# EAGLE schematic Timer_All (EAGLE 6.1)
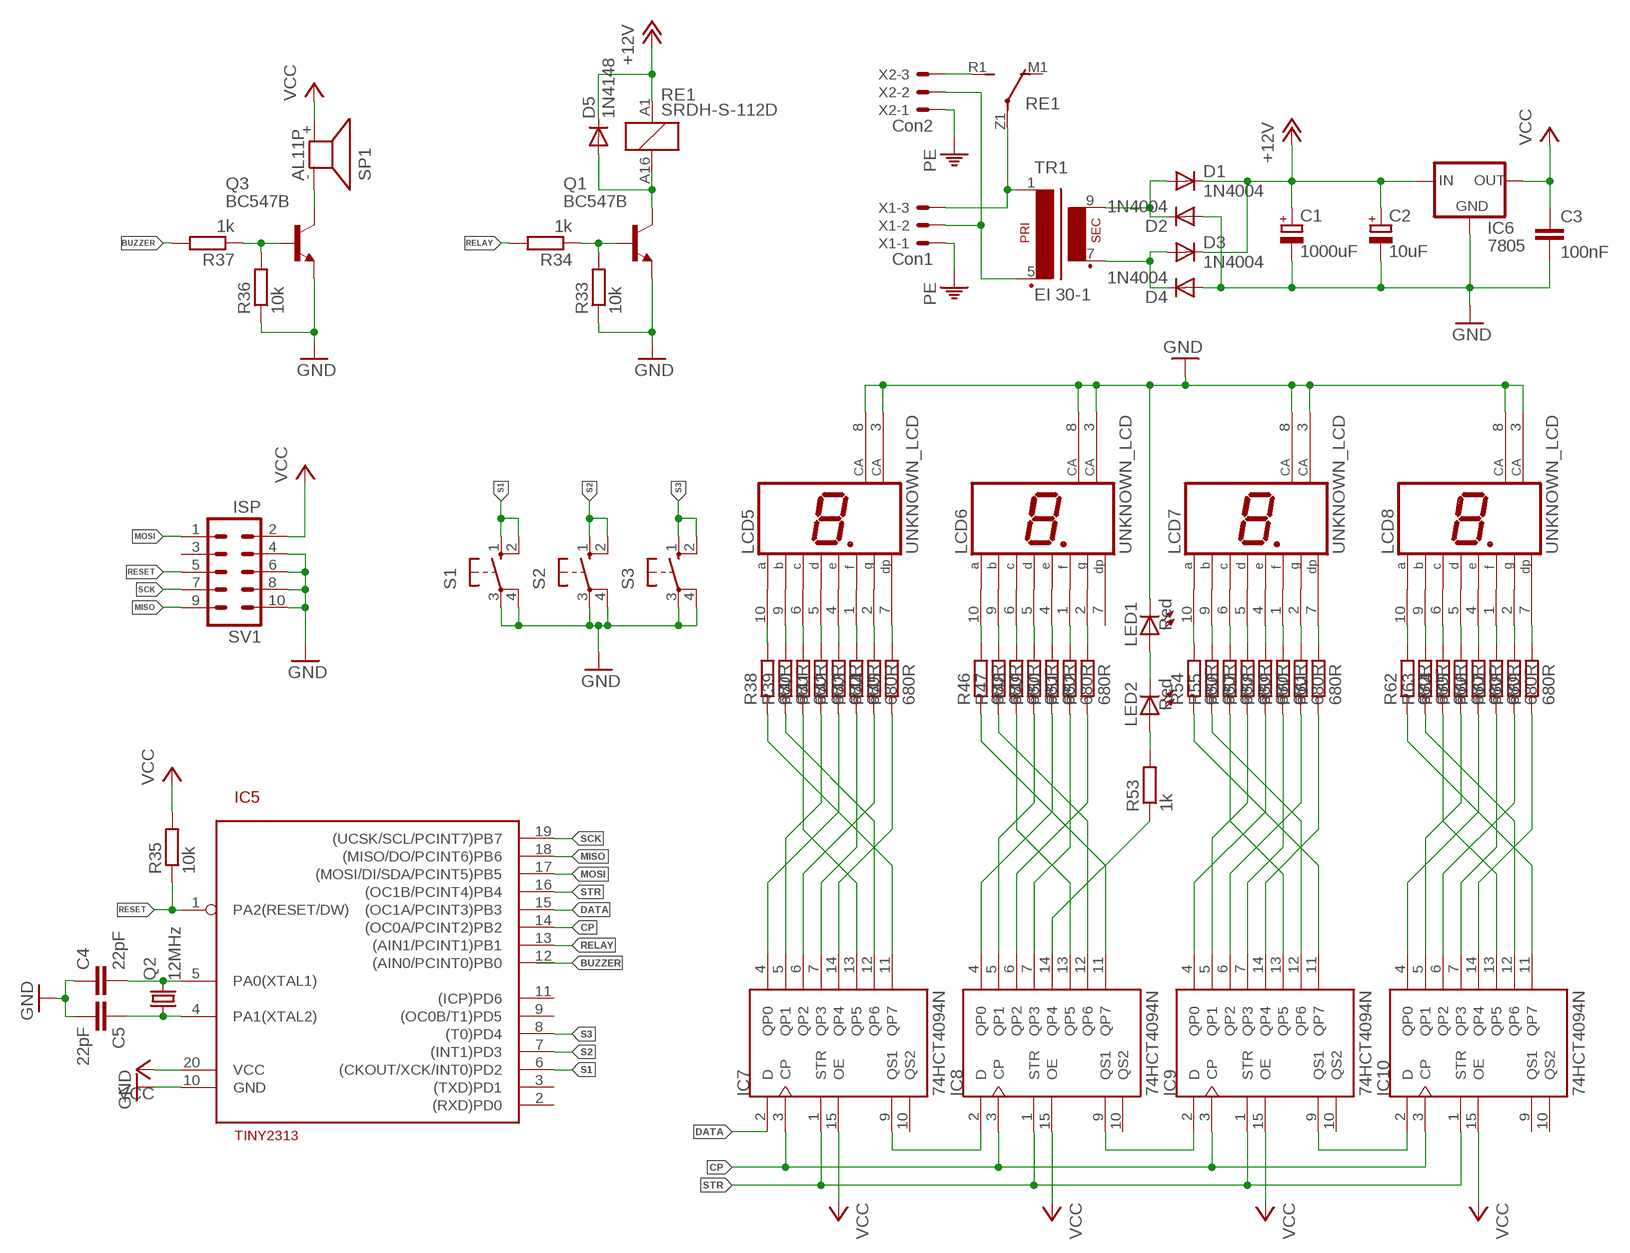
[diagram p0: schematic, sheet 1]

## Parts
C1  1000uF  CPOL-EUTT5D10  [TT5D10]
C2  10uF  CPOL-EUE2.5-5  [E2,5-5]
C3  100nF  C-EU050-025X075  [C050-025X075]
C4  22pF  C-EU025-025X050  [C025-025X050]
C5  22pF  C-EU025-025X050  [C025-025X050]
D1  1N4004  [DO41-10]
D2  1N4004  [DO41-10]
D3  1N4004  [DO41-10]
D4  1N4004  [DO41-10]
D5  1N4148  1N4148DO35-10  [DO35-10]
IC5  TINY2313  [DIL20]
IC6  7805  78XXL  [78XXL]
IC7  74HCT4094N  [DIL16]
IC8  74HCT4094N  [DIL16]
IC9  74HCT4094N  [DIL16]
IC10  74HCT4094N  [DIL16]
LCD5  UNKNOWN_LCD  [CA-MOJ]
LCD6  UNKNOWN_LCD  [CA-MOJ]
LCD7  UNKNOWN_LCD  [CA-MOJ]
LCD8  UNKNOWN_LCD  [CA-MOJ]
LED1  Red  LED3MM  [LED3MM]
LED2  Red  LED3MM  [LED3MM]
Q1  BC547B  [TO92]
Q2  12MHz  CRYSTALHC49S  [HC49/S]
Q3  BC547B  [TO92]
R33  10k  R-EU_0207/10  [0207/10]
R34  1k  R-EU_0207/10  [0207/10]
R35  10k  R-EU_0207/10  [0207/10]
R36  10k  R-EU_0207/10  [0207/10]
R37  1k  R-EU_0207/10  [0207/10]
R38  680R  R-EU_R0805  [R0805]
R39  680R  R-EU_R0805  [R0805]
R40  680R  R-EU_R0805  [R0805]
R41  680R  R-EU_R0805  [R0805]
R42  680R  R-EU_R0805  [R0805]
R43  680R  R-EU_R0805  [R0805]
R44  680R  R-EU_R0805  [R0805]
R45  680R  R-EU_R0805  [R0805]
R46  680R  R-EU_R0805  [R0805]
R47  680R  R-EU_R0805  [R0805]
R48  680R  R-EU_R0805  [R0805]
R49  680R  R-EU_R0805  [R0805]
R50  680R  R-EU_R0805  [R0805]
R51  680R  R-EU_R0805  [R0805]
R52  680R  R-EU_R0805  [R0805]
R53  1k  R-EU_0207/10  [0207/10]
R54  680R  R-EU_R0805  [R0805]
R55  680R  R-EU_R0805  [R0805]
R56  680R  R-EU_R0805  [R0805]
R57  680R  R-EU_R0805  [R0805]
R58  680R  R-EU_R0805  [R0805]
R59  680R  R-EU_R0805  [R0805]
R60  680R  R-EU_R0805  [R0805]
R61  680R  R-EU_R0805  [R0805]
R62  680R  R-EU_R0805  [R0805]
R63  680R  R-EU_R0805  [R0805]
R64  680R  R-EU_R0805  [R0805]
R65  680R  R-EU_R0805  [R0805]
R66  680R  R-EU_R0805  [R0805]
R67  680R  R-EU_R0805  [R0805]
R68  680R  R-EU_R0805  [R0805]
R69  680R  R-EU_R0805  [R0805]
RE1  SRDH-S-112D  [SRDH-S-112D]
S1  10-XX  [B3F-10XX]
S2  10-XX  [B3F-10XX]
S3  10-XX  [B3F-10XX]
SP1  AL11P  [AL11P]
SV1  ISP  ML10  [ML10]
TR1  EI 30-1  EI30-1  [EI30-1]
X1  Con1  KK-156-3  [KK-156-3]
X2  Con2  KK-156-3  [KK-156-3]

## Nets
+12V: C1.+ C2.+ D1.C D3.C D5.C IC6.IN RE1.A1
BUZZER: R37.2
CP: IC7.3(CP) IC8.3(CP) IC9.3(CP) IC10.3(CP)
DATA: IC7.2(D)
GND: C1.- C2.- C3.2 C4.1 C5.2 D2.A D4.A IC5.10(GND) IC6.GND LCD5.3(CA) LCD5.8(CA) LCD6.3(CA) LCD6.8(CA) LCD7.3(CA) LCD7.8(CA) LCD8.3(CA) LCD8.8(CA) LED1.K(C) Q1.1(E) Q3.1(E) R33.1 R36.1 S1.3(P) S1.4(P1) S2.3(P) S2.4(P1) S3.3(P) S3.4(P1) SV1.4 SV1.6 SV1.8 SV1.10
MISO: IC5.18((MISO/DO/PCINT6)PB6) SV1.9
MOSI: IC5.17((MOSI/DI/SDA/PCINT5)PB5) SV1.1
N$65: RE1.Z1(P) TR1.1 X1.3
N$69: TR1.5(P2) X1.2 X2.2
N$70: D1.A D2.C TR1.9(S4)
N$71: D3.A D4.C TR1.7(S3)
N$72: RE1.R1(S) X2.3
N$73: Q1.2(B) R33.2 R34.1
N$74: D5.A Q1.3(C) RE1.A16
N$75: LCD5.10(A) R38.2
N$76: C4.2 IC5.5(PA0(XTAL1)) Q2.2
N$77: C5.1 IC5.4(PA1(XTAL2)) Q2.1
N$78: Q3.2(B) R36.2 R37.1
N$79: Q3.3(C) SP1.-
N$80: LCD5.9(B) R39.2
N$81: LCD5.6(C) R40.2
N$82: LCD5.5(D) R41.2
N$83: LCD5.4(E) R42.2
N$84: LCD5.1(F) R43.2
N$85: LCD5.2(G) R44.2
N$86: LCD5.7(DP) R45.2
N$87: LCD6.2(G) R52.2
N$88: LCD6.1(F) R51.2
N$89: LCD6.4(E) R50.2
N$90: LCD6.5(D) R49.2
N$91: LCD6.6(C) R48.2
N$92: LCD6.9(B) R47.2
N$93: LCD6.10(A) R46.2
N$94: LCD7.10(A) R54.2
N$95: LCD7.9(B) R55.2
N$96: LCD7.6(C) R56.2
N$97: LCD7.5(D) R57.2
N$98: LCD7.4(E) R58.2
N$99: LCD7.1(F) R59.2
N$100: LCD7.2(G) R60.2
N$101: LCD7.7(DP) R61.2
N$102: LCD8.10(A) R62.2
N$103: LCD8.9(B) R63.2
N$104: LCD8.6(C) R64.2
N$105: LCD8.5(D) R65.2
N$106: LCD8.4(E) R66.2
N$107: LCD8.1(F) R67.2
N$108: LCD8.2(G) R68.2
N$109: LCD8.7(DP) R69.2
N$110: IC7.9(QS1) IC8.2(D)
N$111: IC8.9(QS1) IC9.2(D)
N$112: IC9.9(QS1) IC10.2(D)
N$113: IC7.7(QP3) R43.1
N$114: IC7.6(QP2) R44.1
N$115: IC7.4(QP0) R42.1
N$116: IC7.5(QP1) R41.1
N$117: IC7.11(QP7) R38.1
N$118: IC7.12(QP6) R39.1
N$119: IC7.14(QP4) R45.1
N$120: IC7.13(QP5) R40.1
N$121: IC8.11(QP7) R46.1
N$122: IC8.12(QP6) R47.1
N$123: IC8.5(QP1) R49.1
N$124: IC8.4(QP0) R50.1
N$125: IC8.6(QP2) R52.1
N$126: IC8.7(QP3) R51.1
N$127: IC9.12(QP6) R55.1
N$128: IC9.11(QP7) R54.1
N$129: IC9.13(QP5) R56.1
N$130: IC9.5(QP1) R57.1
N$131: IC9.4(QP0) R58.1
N$132: IC9.6(QP2) R60.1
N$133: IC9.7(QP3) R59.1
N$134: IC9.14(QP4) R61.1
N$135: IC10.12(QP6) R63.1
N$136: IC10.11(QP7) R62.1
N$137: IC10.13(QP5) R64.1
N$138: IC10.4(QP0) R66.1
N$139: IC10.6(QP2) R68.1
N$140: IC10.7(QP3) R67.1
N$141: IC10.14(QP4) R69.1
N$142: IC8.13(QP5) R48.1
N$143: LED1.A LED2.K(C)
N$144: LED2.A R53.2
N$145: IC8.14(QP4) R53.1
N$146: IC10.5(QP1) R65.1
PE: X1.1 X2.1
RELAY: R34.2
RESET: IC5.1(PA2(RESET/DW)) R35.1 SV1.5
S1: IC5.6((CKOUT/XCK/INT0)PD2) S1.1(S) S1.2(S1)
S2: IC5.7((INT1)PD3) S2.1(S) S2.2(S1)
S3: IC5.8((T0)PD4) S3.1(S) S3.2(S1)
SCK: IC5.19((UCSK/SCL/PCINT7)PB7) SV1.7
STR: IC7.1(STR) IC8.1(STR) IC9.1(STR) IC10.1(STR)
VCC: C3.1 IC5.20(VCC) IC6.OUT IC7.15(OE) IC8.15(OE) IC9.15(OE) IC10.15(OE) R35.2 SP1.+ SV1.2
Unconnected: IC5.2((RXD)PD0) IC5.3((TXD)PD1) IC5.9((OC0B/T1)PD5) IC5.11((ICP)PD6) IC5.12((AIN0/PCINT0)PB0) IC5.13((AIN1/PCINT1)PB1) IC5.14((OC0A/PCINT2)PB2) IC5.15((OC1A/PCINT3)PB3) IC5.16((OC1B/PCINT4)PB4) IC7.10(QS2) IC8.10(QS2) IC9.10(QS2) IC10.9(QS1) IC10.10(QS2) LCD6.7(DP) RE1.M1(O) SV1.3

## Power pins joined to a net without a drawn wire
GND: IC7.8(GND) IC8.8(GND) IC9.8(GND) IC10.8(GND)
VCC: IC7.16(VCC) IC8.16(VCC) IC9.16(VCC) IC10.16(VCC)

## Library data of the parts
C1 C2 = resistor:CPOL-EU: POLARIZED CAPACITOR, European symbol
C3-C5 = resistor:C-EU: CAPACITOR, European symbol
D1-D4 = diode:1N4004: DIODE
D5 = diode:1N4148: DIODE
IC5 = atmel:TINY2313: 2kB Flash, 20-pin
IC6 = v-reg:78XXL: VOLTAGE REGULATOR
IC7-IC10 = 74xx-eu:74*4094: 8-stage shift-and-store bus register
LCD5-LCD8 = display-hp:UNKNOWN_LCD
LED1 LED2 = led:LED: LED
Q1 Q3 = transistor-npn:BC547*: NPN Transistor
Q2 = crystal:CRYSTAL: CRYSTAL
R33-R69 = resistor:R-EU_: RESISTOR, European symbol
RE1 = relay:SRDH-S-112D: 24V, 10A relay
S1-S3 = switch-omron:10-XX: OMRON SWITCH
SP1 = buzzer:AL11P: SPEAKER
SV1 = con-harting-ml:ML10: HARTING
TR1 = trafo:EI30-1: TRANSFORMER 1 primary winding, 1 secondary winding ERA
X1 X2 = con-molex:KK-156-3: KK 156 HEADER Source: http://www.molex.com/pdm_docs/sd/026604100_sd.pdf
